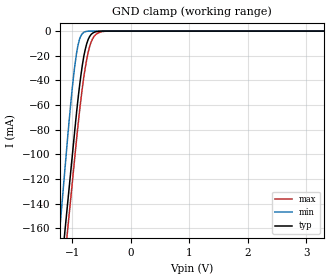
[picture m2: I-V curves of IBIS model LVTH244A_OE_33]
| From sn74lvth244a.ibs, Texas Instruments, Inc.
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[Model]   LVTH244A_OE_33
Model_type  Input
Vinl=0.8
Vinh=2.0
| variable   typ   min   max
C_comp   4.05pF   3.22pF   5.45pF
[Temperature Range]   40   -40   100
| Ambient temperature   25   -40   85
[Voltage range]   3.3   3   3.6
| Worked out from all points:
|   GND clamp passes 1 mA (typ) near -0.62 V on its own axis
[GND Clamp]
| LVTH244A_OE_33
|   Voltage   I(typ)   I(min)   I(max)
-5.5V     -2.407A    -2.647A    -2.408A
-1.22V    -209.3mA   -166mA     -230.3mA
-1.205V   -202mA     -157.5mA   -223mA
-1.125V   -163.1mA   -113mA     -184.4mA
-1.075V   -138.8mA   -85.24mA   -160.3mA
-975mV    -90.17mA   -36.12mA   -112.1mA
-900mV    -55.28mA   -11.44mA   -76.59mA
-825mV    -27.42mA   -1.98mA    -45.77mA
-775mV    -14.64mA   -464.8uA   -29.48mA
-650mV    -1.684mA   -2.076uA   -6.172mA
-395mV    -1.224uA   -43.32pA   -35.83uA
3.3V      16.15pA    8.657pA    1.272nA
